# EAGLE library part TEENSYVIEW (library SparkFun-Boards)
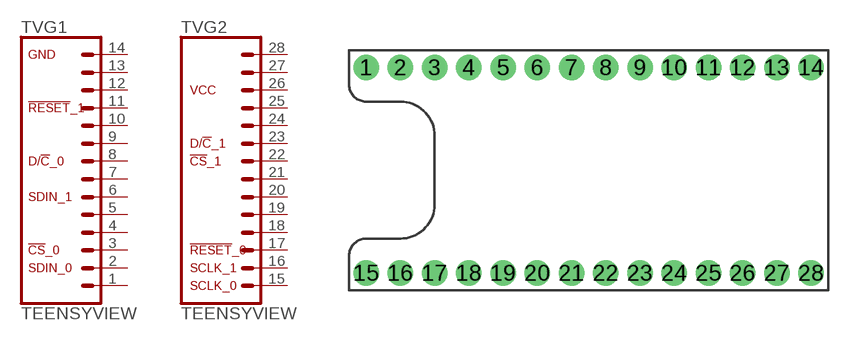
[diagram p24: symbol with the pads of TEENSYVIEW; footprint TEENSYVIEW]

Designator prefix TV; gates G1=TEENSYVIEW_1 G2=TEENSYVIEW_2

## TEENSYVIEW  [TEENSYVIEW]
1  G1:1  pas
2  G1:2  pas
3  G1:3  pas
4  G1:4  pas
5  G1:5  pas
6  G1:6  pas
7  G1:7  pas
8  G1:8  pas
9  G1:9  pas
10  G1:10  pas
11  G1:11  pas
12  G1:12  pas
13  G1:13  pas
14  G1:14  pas
15  G2:1  pas
16  G2:2  pas
17  G2:3  pas
18  G2:4  pas
19  G2:5  pas
20  G2:6  pas
21  G2:7  pas
22  G2:8  pas
23  G2:9  pas
24  G2:10  pas
25  G2:11  pas
26  G2:12  pas
27  G2:13  pas
28  G2:14  pas

## Footprint TEENSYVIEW (pad centres in mm)
drill 1.016 pad 1.88: 1 1.27,16.51; 2 3.81,16.51; 3 6.35,16.51; 4 8.89,16.51; 5 11.43,16.51; 6 13.97,16.51; 7 16.51,16.51; 8 19.05,16.51; 9 21.59,16.51; 10 24.13,16.51; 11 26.67,16.51; 12 29.21,16.51; 13 31.75,16.51; 14 34.29,16.51; 15 1.27,1.27; 16 3.81,1.27; 17 6.35,1.27; 18 8.89,1.27; 19 11.43,1.27; 20 13.97,1.27; 21 16.51,1.27; 22 19.05,1.27; 23 21.59,1.27; 24 24.13,1.27; 25 26.67,1.27; 26 29.21,1.27; 27 31.75,1.27; 28 34.29,1.27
